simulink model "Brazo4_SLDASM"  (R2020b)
settings: Solver=VariableStepAuto  StartTime=0.0  StopTime=20  RelTol=1e-3
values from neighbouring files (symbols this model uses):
  q = [q 0]    [robotSimulation.m]    (also in robotSimulationWithConstraints.m = [q' 0])
undefined symbols (not defined in the file or in its folder): deg, kg, m, N, rad, s, X, Y, Z
libraries: sm_lib x118, nesl_utility x17, pid_lib x4
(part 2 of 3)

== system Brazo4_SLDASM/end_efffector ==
  Inertia : sm_lib/Body Elements/Inertia  InertiaType=Custom  Mass=1.4886  MassUnits=kg  CenterOfMass=[0, 0, 0]  CenterOfMassUnits=m  MomentsOfInertia=[0.00086527, 0.00086527, 0.0015073]  MomentsOfInertiaUnits=kg*m^2  ProductsOfInertia=[-1.4429e-20, -5.8421e-20, 3.3881e-21]  ProductsOfInertiaUnits=kg*m^2  GraphicType=None  MarkerShape=Inertia  MarkerSize=20  GraphicVisPropType=SimpleVisualProperties  GraphicDiffuseColor=[0.5 0.5 0.5]  GraphicSpecularColor=[0.5 0.5 0.5 1.0]  GraphicAmbientColor=[0.15 0.15 0.15 1.0]  GraphicEmissiveColor=[0.0 0.0 0.0 1.0]  GraphicShininess=75  GraphicOpacity=1.0
  InertiaOriginTransform : sm_lib/Frames and Transforms/Rigid Transform  TranslationMethod=Cartesian  TranslationStandardOffset=0  TranslationLengthUnit=m  TranslationStandardAxis=+Z  TranslationCartesianOffset=[5.5511e-17, -3.4694e-18, -0.015]  TranslationROffset=0  TranslationROffsetUnits=m  TranslationZOffset=0  TranslationZOffsetUnits=m  TranslationThetaOffset=0  TranslationThetaOffsetUnits=deg  RotationMethod=RotationSequence  RotationAngleUnits=deg  RotationStandardAxis=+Z  RotationAngle=0.0  RotationArbitraryAxis=[0 0 1]  FollAlignAxisA=+X  BaseAlignAxisA=+Y  FollAlignAxisB=+Y  BaseAlignAxisB=+Z  RotationSequenceAxes=BaseAxes  RotationSequence=XYZ  RotationSequenceAngles=[0, 0, 0]  RotationSequenceAnglesUnits=rad  RotationMatrix=[1 0 0; 0 1 0; 0 0 1]
  ReferenceFrame : sm_lib/Frames and Transforms/Reference Frame
  Visual : sm_lib/Body Elements/File Solid  ExtGeomFileName=Brazo4_SLDASM/meshes/end_efffector.STL  UnitType=Custom  ExtGeomFileUnits=m  StepReaderType=HEX  ExportConvexHullGeometry=off  InertiaType=Custom  Mass=0  MassUnits=kg  CenterOfMass=[0, 0, 0]  CenterOfMassUnits=m  MomentsOfInertia=[0, 0, 0]  MomentsOfInertiaUnits=kg*m^2  ProductsOfInertia=[0, 0, 0]  ProductsOfInertiaUnits=kg*m^2  BasedOnType=DensityFromFile  Density=1000  DensityUnits=kg/m^3  DoExposeReferenceFrame=on  SerializedFrames=<Frames/>  GraphicType=FromGeometry  MarkerShape=Sphere  MarkerSize=10  GraphicVisPropType=SimpleVisualProperties  GraphicDiffuseColor=[0.77647, 0.75686, 0.73725]  GraphicSpecularColor=[0.5 0.5 0.5 1.0]  GraphicAmbientColor=[0.15 0.15 0.15 1.0]  GraphicEmissiveColor=[0.0 0.0 0.0 1.0]  GraphicShininess=75  GraphicOpacity=1
  VisualOriginTransform : sm_lib/Frames and Transforms/Rigid Transform  TranslationMethod=Cartesian  TranslationStandardOffset=0  TranslationLengthUnit=m  TranslationStandardAxis=+Z  TranslationCartesianOffset=[0, 0, 0]  TranslationROffset=0  TranslationROffsetUnits=m  TranslationZOffset=0  TranslationZOffsetUnits=m  TranslationThetaOffset=0  TranslationThetaOffsetUnits=deg  RotationMethod=RotationSequence  RotationAngleUnits=deg  RotationStandardAxis=+Z  RotationAngle=0.0  RotationArbitraryAxis=[0 0 1]  FollAlignAxisA=+X  BaseAlignAxisA=+Y  FollAlignAxisB=+Y  BaseAlignAxisB=+Z  RotationSequenceAxes=BaseAxes  RotationSequence=XYZ  RotationSequenceAngles=[0, 0, 0]  RotationSequenceAnglesUnits=rad  RotationMatrix=[1 0 0; 0 1 0; 0 0 1]
  F : PMIOPort  Side=Left
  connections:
  Inertia/RConn1 -- InertiaOriginTransform/RConn1
  ReferenceFrame/RConn1 -- InertiaOriginTransform/LConn1 -- VisualOriginTransform/LConn1 -- F/RConn1
  Visual/RConn1 -- VisualOriginTransform/RConn1

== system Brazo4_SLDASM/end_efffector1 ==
  Inertia : sm_lib/Body Elements/Inertia  InertiaType=Custom  Mass=1.4886  MassUnits=kg  CenterOfMass=[0, 0, 0]  CenterOfMassUnits=m  MomentsOfInertia=[0.00086527, 0.00086527, 0.0015073]  MomentsOfInertiaUnits=kg*m^2  ProductsOfInertia=[-1.4429e-20, -5.8421e-20, 3.3881e-21]  ProductsOfInertiaUnits=kg*m^2  GraphicType=None  MarkerShape=Inertia  MarkerSize=20  GraphicVisPropType=SimpleVisualProperties  GraphicDiffuseColor=[0.5 0.5 0.5]  GraphicSpecularColor=[0.5 0.5 0.5 1.0]  GraphicAmbientColor=[0.15 0.15 0.15 1.0]  GraphicEmissiveColor=[0.0 0.0 0.0 1.0]  GraphicShininess=75  GraphicOpacity=1.0
  InertiaOriginTransform : sm_lib/Frames and Transforms/Rigid Transform  TranslationMethod=Cartesian  TranslationStandardOffset=0  TranslationLengthUnit=m  TranslationStandardAxis=+Z  TranslationCartesianOffset=[5.5511e-17, -3.4694e-18, -0.015]  TranslationROffset=0  TranslationROffsetUnits=m  TranslationZOffset=0  TranslationZOffsetUnits=m  TranslationThetaOffset=0  TranslationThetaOffsetUnits=deg  RotationMethod=RotationSequence  RotationAngleUnits=deg  RotationStandardAxis=+Z  RotationAngle=0.0  RotationArbitraryAxis=[0 0 1]  FollAlignAxisA=+X  BaseAlignAxisA=+Y  FollAlignAxisB=+Y  BaseAlignAxisB=+Z  RotationSequenceAxes=BaseAxes  RotationSequence=XYZ  RotationSequenceAngles=[0, 0, 0]  RotationSequenceAnglesUnits=rad  RotationMatrix=[1 0 0; 0 1 0; 0 0 1]
  ReferenceFrame : sm_lib/Frames and Transforms/Reference Frame
  Visual : sm_lib/Body Elements/File Solid  ExtGeomFileName=Brazo4_SLDASM/meshes/end_efffector.STL  UnitType=Custom  ExtGeomFileUnits=m  StepReaderType=HEX  ExportConvexHullGeometry=off  InertiaType=Custom  Mass=0  MassUnits=kg  CenterOfMass=[0, 0, 0]  CenterOfMassUnits=m  MomentsOfInertia=[0, 0, 0]  MomentsOfInertiaUnits=kg*m^2  ProductsOfInertia=[0, 0, 0]  ProductsOfInertiaUnits=kg*m^2  BasedOnType=DensityFromFile  Density=1000  DensityUnits=kg/m^3  DoExposeReferenceFrame=on  SerializedFrames=<Frames/>  GraphicType=FromGeometry  MarkerShape=Sphere  MarkerSize=10  GraphicVisPropType=SimpleVisualProperties  GraphicDiffuseColor=[0.77647, 0.75686, 0.73725]  GraphicSpecularColor=[0.5 0.5 0.5 1.0]  GraphicAmbientColor=[0.15 0.15 0.15 1.0]  GraphicEmissiveColor=[0.0 0.0 0.0 1.0]  GraphicShininess=75  GraphicOpacity=1
  VisualOriginTransform : sm_lib/Frames and Transforms/Rigid Transform  TranslationMethod=Cartesian  TranslationStandardOffset=0  TranslationLengthUnit=m  TranslationStandardAxis=+Z  TranslationCartesianOffset=[0, 0, 0]  TranslationROffset=0  TranslationROffsetUnits=m  TranslationZOffset=0  TranslationZOffsetUnits=m  TranslationThetaOffset=0  TranslationThetaOffsetUnits=deg  RotationMethod=RotationSequence  RotationAngleUnits=deg  RotationStandardAxis=+Z  RotationAngle=0.0  RotationArbitraryAxis=[0 0 1]  FollAlignAxisA=+X  BaseAlignAxisA=+Y  FollAlignAxisB=+Y  BaseAlignAxisB=+Z  RotationSequenceAxes=BaseAxes  RotationSequence=XYZ  RotationSequenceAngles=[0, 0, 0]  RotationSequenceAnglesUnits=rad  RotationMatrix=[1 0 0; 0 1 0; 0 0 1]
  F : PMIOPort  Side=Left
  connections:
  Inertia/RConn1 -- InertiaOriginTransform/RConn1
  ReferenceFrame/RConn1 -- InertiaOriginTransform/LConn1 -- VisualOriginTransform/LConn1 -- F/RConn1
  Visual/RConn1 -- VisualOriginTransform/RConn1

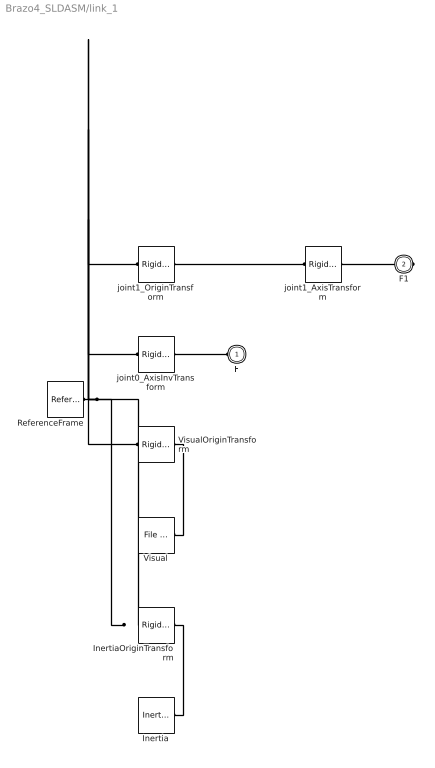
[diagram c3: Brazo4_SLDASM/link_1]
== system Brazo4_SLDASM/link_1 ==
  Inertia : sm_lib/Body Elements/Inertia  InertiaType=Custom  Mass=40.085  MassUnits=kg  CenterOfMass=[0, 0, 0]  CenterOfMassUnits=m  MomentsOfInertia=[0.14011, 0.15124, 0.16589]  MomentsOfInertiaUnits=kg*m^2  ProductsOfInertia=[-5.1752e-17, 1.3296e-17, 1.589e-18]  ProductsOfInertiaUnits=kg*m^2  GraphicType=None  MarkerShape=Inertia  MarkerSize=20  GraphicVisPropType=SimpleVisualProperties  GraphicDiffuseColor=[0.5 0.5 0.5]  GraphicSpecularColor=[0.5 0.5 0.5 1.0]  GraphicAmbientColor=[0.15 0.15 0.15 1.0]  GraphicEmissiveColor=[0.0 0.0 0.0 1.0]  GraphicShininess=75  GraphicOpacity=1.0
  InertiaOriginTransform : sm_lib/Frames and Transforms/Rigid Transform  TranslationMethod=Cartesian  TranslationStandardOffset=0  TranslationLengthUnit=m  TranslationStandardAxis=+Z  TranslationCartesianOffset=[2.7731e-17, 2.4685e-06, 0.28325]  TranslationROffset=0  TranslationROffsetUnits=m  TranslationZOffset=0  TranslationZOffsetUnits=m  TranslationThetaOffset=0  TranslationThetaOffsetUnits=deg  RotationMethod=RotationSequence  RotationAngleUnits=deg  RotationStandardAxis=+Z  RotationAngle=0.0  RotationArbitraryAxis=[0 0 1]  FollAlignAxisA=+X  BaseAlignAxisA=+Y  FollAlignAxisB=+Y  BaseAlignAxisB=+Z  RotationSequenceAxes=BaseAxes  RotationSequence=XYZ  RotationSequenceAngles=[0, 0, 0]  RotationSequenceAnglesUnits=rad  RotationMatrix=[1 0 0; 0 1 0; 0 0 1]
  ReferenceFrame : sm_lib/Frames and Transforms/Reference Frame
  Visual : sm_lib/Body Elements/File Solid  ExtGeomFileName=Brazo4_SLDASM/meshes/link_1.STL  UnitType=Custom  ExtGeomFileUnits=m  StepReaderType=HEX  ExportConvexHullGeometry=off  InertiaType=Custom  Mass=0  MassUnits=kg  CenterOfMass=[0, 0, 0]  CenterOfMassUnits=m  MomentsOfInertia=[0, 0, 0]  MomentsOfInertiaUnits=kg*m^2  ProductsOfInertia=[0, 0, 0]  ProductsOfInertiaUnits=kg*m^2  BasedOnType=DensityFromFile  Density=1000  DensityUnits=kg/m^3  DoExposeReferenceFrame=on  SerializedFrames=<Frames/>  GraphicType=FromGeometry  MarkerShape=Sphere  MarkerSize=10  GraphicVisPropType=SimpleVisualProperties  GraphicDiffuseColor=[0.77647, 0.75686, 0.73725]  GraphicSpecularColor=[0.5 0.5 0.5 1.0]  GraphicAmbientColor=[0.15 0.15 0.15 1.0]  GraphicEmissiveColor=[0.0 0.0 0.0 1.0]  GraphicShininess=75  GraphicOpacity=1
  VisualOriginTransform : sm_lib/Frames and Transforms/Rigid Transform  TranslationMethod=Cartesian  TranslationStandardOffset=0  TranslationLengthUnit=m  TranslationStandardAxis=+Z  TranslationCartesianOffset=[0, 0, 0]  TranslationROffset=0  TranslationROffsetUnits=m  TranslationZOffset=0  TranslationZOffsetUnits=m  TranslationThetaOffset=0  TranslationThetaOffsetUnits=deg  RotationMethod=RotationSequence  RotationAngleUnits=deg  RotationStandardAxis=+Z  RotationAngle=0.0  RotationArbitraryAxis=[0 0 1]  FollAlignAxisA=+X  BaseAlignAxisA=+Y  FollAlignAxisB=+Y  BaseAlignAxisB=+Z  RotationSequenceAxes=BaseAxes  RotationSequence=XYZ  RotationSequenceAngles=[0, 0, 0]  RotationSequenceAnglesUnits=rad  RotationMatrix=[1 0 0; 0 1 0; 0 0 1]
  joint0_AxisInvTransform : sm_lib/Frames and Transforms/Rigid Transform  TranslationMethod=Cartesian  TranslationStandardOffset=0  TranslationLengthUnit=m  TranslationStandardAxis=+Z  TranslationCartesianOffset=[0, 0, 0]  TranslationROffset=0  TranslationROffsetUnits=m  TranslationZOffset=0  TranslationZOffsetUnits=m  TranslationThetaOffset=0  TranslationThetaOffsetUnits=deg  RotationMethod=ArbitraryAxis  RotationAngleUnits=rad  RotationStandardAxis=+Z  RotationAngle=0  RotationArbitraryAxis=[1, 0, 0]  FollAlignAxisA=+X  BaseAlignAxisA=+Y  FollAlignAxisB=+Y  BaseAlignAxisB=+Z  RotationSequenceAxes=FollowerAxes  RotationSequence=XYX  RotationSequenceAngles=[0 0 0]  RotationSequenceAnglesUnits=deg  RotationMatrix=[1 0 0; 0 1 0; 0 0 1]
  joint1_AxisTransform : sm_lib/Frames and Transforms/Rigid Transform  TranslationMethod=Cartesian  TranslationStandardOffset=0  TranslationLengthUnit=m  TranslationStandardAxis=+Z  TranslationCartesianOffset=[0, 0, 0]  TranslationROffset=0  TranslationROffsetUnits=m  TranslationZOffset=0  TranslationZOffsetUnits=m  TranslationThetaOffset=0  TranslationThetaOffsetUnits=deg  RotationMethod=ArbitraryAxis  RotationAngleUnits=rad  RotationStandardAxis=+Z  RotationAngle=0  RotationArbitraryAxis=[1, 0, 0]  FollAlignAxisA=+X  BaseAlignAxisA=+Y  FollAlignAxisB=+Y  BaseAlignAxisB=+Z  RotationSequenceAxes=FollowerAxes  RotationSequence=XYX  RotationSequenceAngles=[0 0 0]  RotationSequenceAnglesUnits=deg  RotationMatrix=[1 0 0; 0 1 0; 0 0 1]
  joint1_OriginTransform : sm_lib/Frames and Transforms/Rigid Transform  TranslationMethod=Cartesian  TranslationStandardOffset=0  TranslationLengthUnit=m  TranslationStandardAxis=+Z  TranslationCartesianOffset=[0, 0, 0.35051]  TranslationROffset=0  TranslationROffsetUnits=m  TranslationZOffset=0  TranslationZOffsetUnits=m  TranslationThetaOffset=0  TranslationThetaOffsetUnits=deg  RotationMethod=RotationSequence  RotationAngleUnits=deg  RotationStandardAxis=+Z  RotationAngle=0.0  RotationArbitraryAxis=[0 0 1]  FollAlignAxisA=+X  BaseAlignAxisA=+Y  FollAlignAxisB=+Y  BaseAlignAxisB=+Z  RotationSequenceAxes=BaseAxes  RotationSequence=XYZ  RotationSequenceAngles=[1.5708, 0, 1.5708]  RotationSequenceAnglesUnits=rad  RotationMatrix=[1 0 0; 0 1 0; 0 0 1]
  F : PMIOPort  Side=Left
  F1 : PMIOPort  Port=2  Side=Right
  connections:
  Inertia/RConn1 -- InertiaOriginTransform/RConn1
  ReferenceFrame/RConn1 -- InertiaOriginTransform/LConn1 -- VisualOriginTransform/LConn1 -- joint0_AxisInvTransform/LConn1 -- joint1_OriginTransform/LConn1
  Visual/RConn1 -- VisualOriginTransform/RConn1
  joint0_AxisInvTransform/RConn1 -- F/RConn1
  joint1_AxisTransform/RConn1 -- F1/RConn1
  joint1_AxisTransform/LConn1 -- joint1_OriginTransform/RConn1

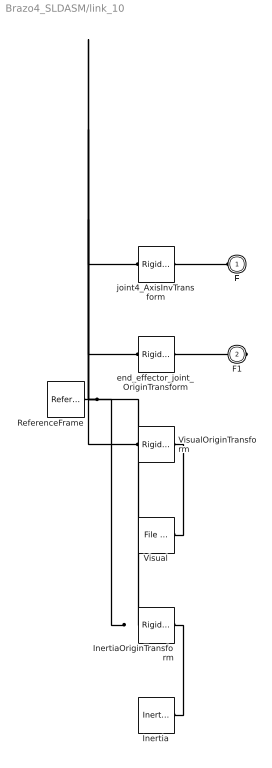
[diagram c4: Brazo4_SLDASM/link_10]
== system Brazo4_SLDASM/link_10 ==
  Inertia : sm_lib/Body Elements/Inertia  InertiaType=Custom  Mass=1.4886  MassUnits=kg  CenterOfMass=[0, 0, 0]  CenterOfMassUnits=m  MomentsOfInertia=[0.00086527, 0.00086527, 0.0015073]  MomentsOfInertiaUnits=kg*m^2  ProductsOfInertia=[-1.5349e-20, -1.2683e-19, -7.4327e-21]  ProductsOfInertiaUnits=kg*m^2  GraphicType=None  MarkerShape=Inertia  MarkerSize=20  GraphicVisPropType=SimpleVisualProperties  GraphicDiffuseColor=[0.5 0.5 0.5]  GraphicSpecularColor=[0.5 0.5 0.5 1.0]  GraphicAmbientColor=[0.15 0.15 0.15 1.0]  GraphicEmissiveColor=[0.0 0.0 0.0 1.0]  GraphicShininess=75  GraphicOpacity=1.0
  InertiaOriginTransform : sm_lib/Frames and Transforms/Rigid Transform  TranslationMethod=Cartesian  TranslationStandardOffset=0  TranslationLengthUnit=m  TranslationStandardAxis=+Z  TranslationCartesianOffset=[1.1102e-16, -1.5173e-17, 0.08550000000000001]  TranslationROffset=0  TranslationROffsetUnits=m  TranslationZOffset=0  TranslationZOffsetUnits=m  TranslationThetaOffset=0  TranslationThetaOffsetUnits=deg  RotationMethod=RotationSequence  RotationAngleUnits=deg  RotationStandardAxis=+Z  RotationAngle=0.0  RotationArbitraryAxis=[0 0 1]  FollAlignAxisA=+X  BaseAlignAxisA=+Y  FollAlignAxisB=+Y  BaseAlignAxisB=+Z  RotationSequenceAxes=BaseAxes  RotationSequence=XYZ  RotationSequenceAngles=[0, 0, 0]  RotationSequenceAnglesUnits=rad  RotationMatrix=[1 0 0; 0 1 0; 0 0 1]
  ReferenceFrame : sm_lib/Frames and Transforms/Reference Frame
  Visual : sm_lib/Body Elements/File Solid  ExtGeomFileName=Brazo4_SLDASM/meshes/link_5.STL  UnitType=Custom  ExtGeomFileUnits=m  StepReaderType=HEX  ExportConvexHullGeometry=off  InertiaType=Custom  Mass=0  MassUnits=kg  CenterOfMass=[0, 0, 0]  CenterOfMassUnits=m  MomentsOfInertia=[0, 0, 0]  MomentsOfInertiaUnits=kg*m^2  ProductsOfInertia=[0, 0, 0]  ProductsOfInertiaUnits=kg*m^2  BasedOnType=DensityFromFile  Density=1000  DensityUnits=kg/m^3  DoExposeReferenceFrame=on  SerializedFrames=<Frames/>  GraphicType=FromGeometry  MarkerShape=Sphere  MarkerSize=10  GraphicVisPropType=SimpleVisualProperties  GraphicDiffuseColor=[0.77647, 0.75686, 0.73725]  GraphicSpecularColor=[0.5 0.5 0.5 1.0]  GraphicAmbientColor=[0.15 0.15 0.15 1.0]  GraphicEmissiveColor=[0.0 0.0 0.0 1.0]  GraphicShininess=75  GraphicOpacity=1
  VisualOriginTransform : sm_lib/Frames and Transforms/Rigid Transform  TranslationMethod=Cartesian  TranslationStandardOffset=0  TranslationLengthUnit=m  TranslationStandardAxis=+Z  TranslationCartesianOffset=[0, 0, 0]  TranslationROffset=0  TranslationROffsetUnits=m  TranslationZOffset=0  TranslationZOffsetUnits=m  TranslationThetaOffset=0  TranslationThetaOffsetUnits=deg  RotationMethod=RotationSequence  RotationAngleUnits=deg  RotationStandardAxis=+Z  RotationAngle=0.0  RotationArbitraryAxis=[0 0 1]  FollAlignAxisA=+X  BaseAlignAxisA=+Y  FollAlignAxisB=+Y  BaseAlignAxisB=+Z  RotationSequenceAxes=BaseAxes  RotationSequence=XYZ  RotationSequenceAngles=[0, 0, 0]  RotationSequenceAnglesUnits=rad  RotationMatrix=[1 0 0; 0 1 0; 0 0 1]
  end_effector_joint_OriginTransform : sm_lib/Frames and Transforms/Rigid Transform  TranslationMethod=Cartesian  TranslationStandardOffset=0  TranslationLengthUnit=m  TranslationStandardAxis=+Z  TranslationCartesianOffset=[0, 0, 0.1005]  TranslationROffset=0  TranslationROffsetUnits=m  TranslationZOffset=0  TranslationZOffsetUnits=m  TranslationThetaOffset=0  TranslationThetaOffsetUnits=deg  RotationMethod=RotationSequence  RotationAngleUnits=deg  RotationStandardAxis=+Z  RotationAngle=0.0  RotationArbitraryAxis=[0 0 1]  FollAlignAxisA=+X  BaseAlignAxisA=+Y  FollAlignAxisB=+Y  BaseAlignAxisB=+Z  RotationSequenceAxes=BaseAxes  RotationSequence=XYZ  RotationSequenceAngles=[0, 0, 0.045381]  RotationSequenceAnglesUnits=rad  RotationMatrix=[1 0 0; 0 1 0; 0 0 1]
  joint4_AxisInvTransform : sm_lib/Frames and Transforms/Rigid Transform  TranslationMethod=Cartesian  TranslationStandardOffset=0  TranslationLengthUnit=m  TranslationStandardAxis=+Z  TranslationCartesianOffset=[0, 0, 0]  TranslationROffset=0  TranslationROffsetUnits=m  TranslationZOffset=0  TranslationZOffsetUnits=m  TranslationThetaOffset=0  TranslationThetaOffsetUnits=deg  RotationMethod=ArbitraryAxis  RotationAngleUnits=rad  RotationStandardAxis=+Z  RotationAngle=0  RotationArbitraryAxis=[1, 0, 0]  FollAlignAxisA=+X  BaseAlignAxisA=+Y  FollAlignAxisB=+Y  BaseAlignAxisB=+Z  RotationSequenceAxes=FollowerAxes  RotationSequence=XYX  RotationSequenceAngles=[0 0 0]  RotationSequenceAnglesUnits=deg  RotationMatrix=[1 0 0; 0 1 0; 0 0 1]
  F : PMIOPort  Side=Left
  F1 : PMIOPort  Port=2  Side=Right
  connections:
  Inertia/RConn1 -- InertiaOriginTransform/RConn1
  ReferenceFrame/RConn1 -- InertiaOriginTransform/LConn1 -- VisualOriginTransform/LConn1 -- end_effector_joint_OriginTransform/LConn1 -- joint4_AxisInvTransform/LConn1
  Visual/RConn1 -- VisualOriginTransform/RConn1
  end_effector_joint_OriginTransform/RConn1 -- F1/RConn1
  joint4_AxisInvTransform/RConn1 -- F/RConn1

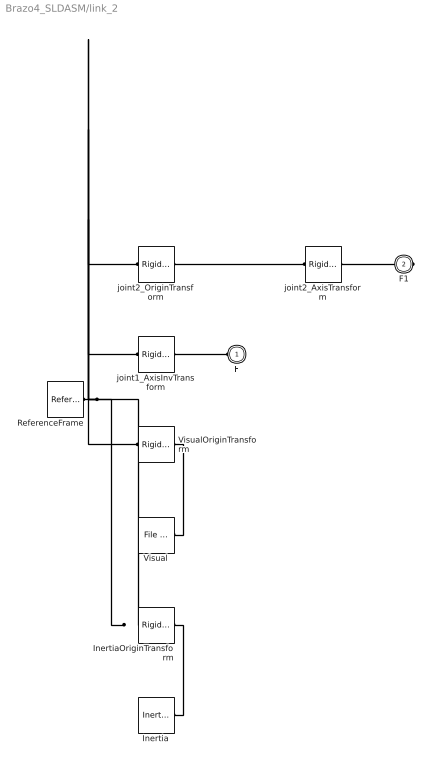
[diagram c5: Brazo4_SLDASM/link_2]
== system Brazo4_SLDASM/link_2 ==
  Inertia : sm_lib/Body Elements/Inertia  InertiaType=Custom  Mass=34.189  MassUnits=kg  CenterOfMass=[0, 0, 0]  CenterOfMassUnits=m  MomentsOfInertia=[0.101, 0.32346, 0.28584]  MomentsOfInertiaUnits=kg*m^2  ProductsOfInertia=[-2.191e-18, 8.7345e-17, 3.6996e-17]  ProductsOfInertiaUnits=kg*m^2  GraphicType=None  MarkerShape=Inertia  MarkerSize=20  GraphicVisPropType=SimpleVisualProperties  GraphicDiffuseColor=[0.5 0.5 0.5]  GraphicSpecularColor=[0.5 0.5 0.5 1.0]  GraphicAmbientColor=[0.15 0.15 0.15 1.0]  GraphicEmissiveColor=[0.0 0.0 0.0 1.0]  GraphicShininess=75  GraphicOpacity=1.0
  InertiaOriginTransform : sm_lib/Frames and Transforms/Rigid Transform  TranslationMethod=Cartesian  TranslationStandardOffset=0  TranslationLengthUnit=m  TranslationStandardAxis=+Z  TranslationCartesianOffset=[0.07391200000000001, 0, -1.2748e-17]  TranslationROffset=0  TranslationROffsetUnits=m  TranslationZOffset=0  TranslationZOffsetUnits=m  TranslationThetaOffset=0  TranslationThetaOffsetUnits=deg  RotationMethod=RotationSequence  RotationAngleUnits=deg  RotationStandardAxis=+Z  RotationAngle=0.0  RotationArbitraryAxis=[0 0 1]  FollAlignAxisA=+X  BaseAlignAxisA=+Y  FollAlignAxisB=+Y  BaseAlignAxisB=+Z  RotationSequenceAxes=BaseAxes  RotationSequence=XYZ  RotationSequenceAngles=[0, 0, 0]  RotationSequenceAnglesUnits=rad  RotationMatrix=[1 0 0; 0 1 0; 0 0 1]
  ReferenceFrame : sm_lib/Frames and Transforms/Reference Frame
  Visual : sm_lib/Body Elements/File Solid  ExtGeomFileName=Brazo4_SLDASM/meshes/link_2.STL  UnitType=Custom  ExtGeomFileUnits=m  StepReaderType=HEX  ExportConvexHullGeometry=off  InertiaType=Custom  Mass=0  MassUnits=kg  CenterOfMass=[0, 0, 0]  CenterOfMassUnits=m  MomentsOfInertia=[0, 0, 0]  MomentsOfInertiaUnits=kg*m^2  ProductsOfInertia=[0, 0, 0]  ProductsOfInertiaUnits=kg*m^2  BasedOnType=DensityFromFile  Density=1000  DensityUnits=kg/m^3  DoExposeReferenceFrame=on  SerializedFrames=<Frames/>  GraphicType=FromGeometry  MarkerShape=Sphere  MarkerSize=10  GraphicVisPropType=SimpleVisualProperties  GraphicDiffuseColor=[0.77647, 0.75686, 0.73725]  GraphicSpecularColor=[0.5 0.5 0.5 1.0]  GraphicAmbientColor=[0.15 0.15 0.15 1.0]  GraphicEmissiveColor=[0.0 0.0 0.0 1.0]  GraphicShininess=75  GraphicOpacity=1
  VisualOriginTransform : sm_lib/Frames and Transforms/Rigid Transform  TranslationMethod=Cartesian  TranslationStandardOffset=0  TranslationLengthUnit=m  TranslationStandardAxis=+Z  TranslationCartesianOffset=[0, 0, 0]  TranslationROffset=0  TranslationROffsetUnits=m  TranslationZOffset=0  TranslationZOffsetUnits=m  TranslationThetaOffset=0  TranslationThetaOffsetUnits=deg  RotationMethod=RotationSequence  RotationAngleUnits=deg  RotationStandardAxis=+Z  RotationAngle=0.0  RotationArbitraryAxis=[0 0 1]  FollAlignAxisA=+X  BaseAlignAxisA=+Y  FollAlignAxisB=+Y  BaseAlignAxisB=+Z  RotationSequenceAxes=BaseAxes  RotationSequence=XYZ  RotationSequenceAngles=[0, 0, 0]  RotationSequenceAnglesUnits=rad  RotationMatrix=[1 0 0; 0 1 0; 0 0 1]
  joint1_AxisInvTransform : sm_lib/Frames and Transforms/Rigid Transform  TranslationMethod=Cartesian  TranslationStandardOffset=0  TranslationLengthUnit=m  TranslationStandardAxis=+Z  TranslationCartesianOffset=[0, 0, 0]  TranslationROffset=0  TranslationROffsetUnits=m  TranslationZOffset=0  TranslationZOffsetUnits=m  TranslationThetaOffset=0  TranslationThetaOffsetUnits=deg  RotationMethod=ArbitraryAxis  RotationAngleUnits=rad  RotationStandardAxis=+Z  RotationAngle=0  RotationArbitraryAxis=[1, 0, 0]  FollAlignAxisA=+X  BaseAlignAxisA=+Y  FollAlignAxisB=+Y  BaseAlignAxisB=+Z  RotationSequenceAxes=FollowerAxes  RotationSequence=XYX  RotationSequenceAngles=[0 0 0]  RotationSequenceAnglesUnits=deg  RotationMatrix=[1 0 0; 0 1 0; 0 0 1]
  joint2_AxisTransform : sm_lib/Frames and Transforms/Rigid Transform  TranslationMethod=Cartesian  TranslationStandardOffset=0  TranslationLengthUnit=m  TranslationStandardAxis=+Z  TranslationCartesianOffset=[0, 0, 0]  TranslationROffset=0  TranslationROffsetUnits=m  TranslationZOffset=0  TranslationZOffsetUnits=m  TranslationThetaOffset=0  TranslationThetaOffsetUnits=deg  RotationMethod=ArbitraryAxis  RotationAngleUnits=rad  RotationStandardAxis=+Z  RotationAngle=0  RotationArbitraryAxis=[1, 0, 0]  FollAlignAxisA=+X  BaseAlignAxisA=+Y  FollAlignAxisB=+Y  BaseAlignAxisB=+Z  RotationSequenceAxes=FollowerAxes  RotationSequence=XYX  RotationSequenceAngles=[0 0 0]  RotationSequenceAnglesUnits=deg  RotationMatrix=[1 0 0; 0 1 0; 0 0 1]
  joint2_OriginTransform : sm_lib/Frames and Transforms/Rigid Transform  TranslationMethod=Cartesian  TranslationStandardOffset=0  TranslationLengthUnit=m  TranslationStandardAxis=+Z  TranslationCartesianOffset=[0.25, 0, 0]  TranslationROffset=0  TranslationROffsetUnits=m  TranslationZOffset=0  TranslationZOffsetUnits=m  TranslationThetaOffset=0  TranslationThetaOffsetUnits=deg  RotationMethod=RotationSequence  RotationAngleUnits=deg  RotationStandardAxis=+Z  RotationAngle=0.0  RotationArbitraryAxis=[0 0 1]  FollAlignAxisA=+X  BaseAlignAxisA=+Y  FollAlignAxisB=+Y  BaseAlignAxisB=+Z  RotationSequenceAxes=BaseAxes  RotationSequence=XYZ  RotationSequenceAngles=[0, 0, 0]  RotationSequenceAnglesUnits=rad  RotationMatrix=[1 0 0; 0 1 0; 0 0 1]
  F : PMIOPort  Side=Left
  F1 : PMIOPort  Port=2  Side=Right
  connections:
  Inertia/RConn1 -- InertiaOriginTransform/RConn1
  ReferenceFrame/RConn1 -- InertiaOriginTransform/LConn1 -- VisualOriginTransform/LConn1 -- joint1_AxisInvTransform/LConn1 -- joint2_OriginTransform/LConn1
  Visual/RConn1 -- VisualOriginTransform/RConn1
  joint1_AxisInvTransform/RConn1 -- F/RConn1
  joint2_AxisTransform/RConn1 -- F1/RConn1
  joint2_AxisTransform/LConn1 -- joint2_OriginTransform/RConn1

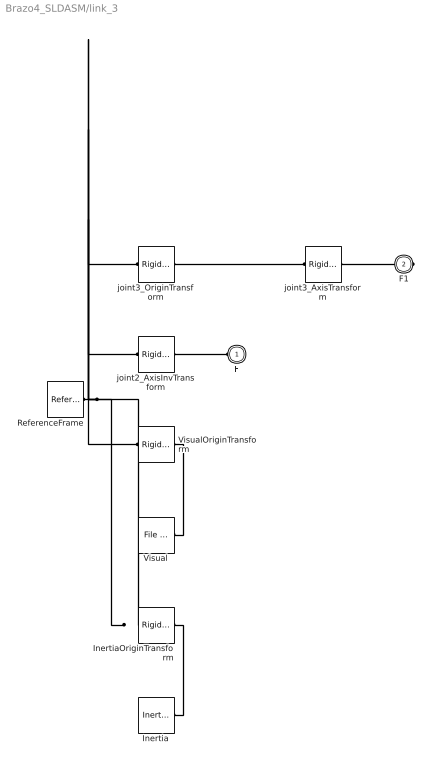
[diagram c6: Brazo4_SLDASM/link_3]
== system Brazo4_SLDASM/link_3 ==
  Inertia : sm_lib/Body Elements/Inertia  InertiaType=Custom  Mass=13.946  MassUnits=kg  CenterOfMass=[0, 0, 0]  CenterOfMassUnits=m  MomentsOfInertia=[0.026465, 0.06281399999999999, 0.054336]  MomentsOfInertiaUnits=kg*m^2  ProductsOfInertia=[-5.1463e-19, 1.9268e-17, 6.4193e-18]  ProductsOfInertiaUnits=kg*m^2  GraphicType=None  MarkerShape=Inertia  MarkerSize=20  GraphicVisPropType=SimpleVisualProperties  GraphicDiffuseColor=[0.5 0.5 0.5]  GraphicSpecularColor=[0.5 0.5 0.5 1.0]  GraphicAmbientColor=[0.15 0.15 0.15 1.0]  GraphicEmissiveColor=[0.0 0.0 0.0 1.0]  GraphicShininess=75  GraphicOpacity=1.0
  InertiaOriginTransform : sm_lib/Frames and Transforms/Rigid Transform  TranslationMethod=Cartesian  TranslationStandardOffset=0  TranslationLengthUnit=m  TranslationStandardAxis=+Z  TranslationCartesianOffset=[0.053841, 0, -3.1131e-17]  TranslationROffset=0  TranslationROffsetUnits=m  TranslationZOffset=0  TranslationZOffsetUnits=m  TranslationThetaOffset=0  TranslationThetaOffsetUnits=deg  RotationMethod=RotationSequence  RotationAngleUnits=deg  RotationStandardAxis=+Z  RotationAngle=0.0  RotationArbitraryAxis=[0 0 1]  FollAlignAxisA=+X  BaseAlignAxisA=+Y  FollAlignAxisB=+Y  BaseAlignAxisB=+Z  RotationSequenceAxes=BaseAxes  RotationSequence=XYZ  RotationSequenceAngles=[0, 0, 0]  RotationSequenceAnglesUnits=rad  RotationMatrix=[1 0 0; 0 1 0; 0 0 1]
  ReferenceFrame : sm_lib/Frames and Transforms/Reference Frame
  Visual : sm_lib/Body Elements/File Solid  ExtGeomFileName=Brazo4_SLDASM/meshes/link_3.STL  UnitType=Custom  ExtGeomFileUnits=m  StepReaderType=HEX  ExportConvexHullGeometry=off  InertiaType=Custom  Mass=0  MassUnits=kg  CenterOfMass=[0, 0, 0]  CenterOfMassUnits=m  MomentsOfInertia=[0, 0, 0]  MomentsOfInertiaUnits=kg*m^2  ProductsOfInertia=[0, 0, 0]  ProductsOfInertiaUnits=kg*m^2  BasedOnType=DensityFromFile  Density=1000  DensityUnits=kg/m^3  DoExposeReferenceFrame=on  SerializedFrames=<Frames/>  GraphicType=FromGeometry  MarkerShape=Sphere  MarkerSize=10  GraphicVisPropType=SimpleVisualProperties  GraphicDiffuseColor=[0.77647, 0.75686, 0.73725]  GraphicSpecularColor=[0.5 0.5 0.5 1.0]  GraphicAmbientColor=[0.15 0.15 0.15 1.0]  GraphicEmissiveColor=[0.0 0.0 0.0 1.0]  GraphicShininess=75  GraphicOpacity=1
  VisualOriginTransform : sm_lib/Frames and Transforms/Rigid Transform  TranslationMethod=Cartesian  TranslationStandardOffset=0  TranslationLengthUnit=m  TranslationStandardAxis=+Z  TranslationCartesianOffset=[0, 0, 0]  TranslationROffset=0  TranslationROffsetUnits=m  TranslationZOffset=0  TranslationZOffsetUnits=m  TranslationThetaOffset=0  TranslationThetaOffsetUnits=deg  RotationMethod=RotationSequence  RotationAngleUnits=deg  RotationStandardAxis=+Z  RotationAngle=0.0  RotationArbitraryAxis=[0 0 1]  FollAlignAxisA=+X  BaseAlignAxisA=+Y  FollAlignAxisB=+Y  BaseAlignAxisB=+Z  RotationSequenceAxes=BaseAxes  RotationSequence=XYZ  RotationSequenceAngles=[0, 0, 0]  RotationSequenceAnglesUnits=rad  RotationMatrix=[1 0 0; 0 1 0; 0 0 1]
  joint2_AxisInvTransform : sm_lib/Frames and Transforms/Rigid Transform  TranslationMethod=Cartesian  TranslationStandardOffset=0  TranslationLengthUnit=m  TranslationStandardAxis=+Z  TranslationCartesianOffset=[0, 0, 0]  TranslationROffset=0  TranslationROffsetUnits=m  TranslationZOffset=0  TranslationZOffsetUnits=m  TranslationThetaOffset=0  TranslationThetaOffsetUnits=deg  RotationMethod=ArbitraryAxis  RotationAngleUnits=rad  RotationStandardAxis=+Z  RotationAngle=0  RotationArbitraryAxis=[1, 0, 0]  FollAlignAxisA=+X  BaseAlignAxisA=+Y  FollAlignAxisB=+Y  BaseAlignAxisB=+Z  RotationSequenceAxes=FollowerAxes  RotationSequence=XYX  RotationSequenceAngles=[0 0 0]  RotationSequenceAnglesUnits=deg  RotationMatrix=[1 0 0; 0 1 0; 0 0 1]
  joint3_AxisTransform : sm_lib/Frames and Transforms/Rigid Transform  TranslationMethod=Cartesian  TranslationStandardOffset=0  TranslationLengthUnit=m  TranslationStandardAxis=+Z  TranslationCartesianOffset=[0, 0, 0]  TranslationROffset=0  TranslationROffsetUnits=m  TranslationZOffset=0  TranslationZOffsetUnits=m  TranslationThetaOffset=0  TranslationThetaOffsetUnits=deg  RotationMethod=ArbitraryAxis  RotationAngleUnits=rad  RotationStandardAxis=+Z  RotationAngle=0  RotationArbitraryAxis=[1, 0, 0]  FollAlignAxisA=+X  BaseAlignAxisA=+Y  FollAlignAxisB=+Y  BaseAlignAxisB=+Z  RotationSequenceAxes=FollowerAxes  RotationSequence=XYX  RotationSequenceAngles=[0 0 0]  RotationSequenceAnglesUnits=deg  RotationMatrix=[1 0 0; 0 1 0; 0 0 1]
  joint3_OriginTransform : sm_lib/Frames and Transforms/Rigid Transform  TranslationMethod=Cartesian  TranslationStandardOffset=0  TranslationLengthUnit=m  TranslationStandardAxis=+Z  TranslationCartesianOffset=[0.16, 0, 0]  TranslationROffset=0  TranslationROffsetUnits=m  TranslationZOffset=0  TranslationZOffsetUnits=m  TranslationThetaOffset=0  TranslationThetaOffsetUnits=deg  RotationMethod=RotationSequence  RotationAngleUnits=deg  RotationStandardAxis=+Z  RotationAngle=0.0  RotationArbitraryAxis=[0 0 1]  FollAlignAxisA=+X  BaseAlignAxisA=+Y  FollAlignAxisB=+Y  BaseAlignAxisB=+Z  RotationSequenceAxes=BaseAxes  RotationSequence=XYZ  RotationSequenceAngles=[0, 0, 0]  RotationSequenceAnglesUnits=rad  RotationMatrix=[1 0 0; 0 1 0; 0 0 1]
  F : PMIOPort  Side=Left
  F1 : PMIOPort  Port=2  Side=Right
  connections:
  Inertia/RConn1 -- InertiaOriginTransform/RConn1
  ReferenceFrame/RConn1 -- InertiaOriginTransform/LConn1 -- VisualOriginTransform/LConn1 -- joint2_AxisInvTransform/LConn1 -- joint3_OriginTransform/LConn1
  Visual/RConn1 -- VisualOriginTransform/RConn1
  joint2_AxisInvTransform/RConn1 -- F/RConn1
  joint3_AxisTransform/RConn1 -- F1/RConn1
  joint3_AxisTransform/LConn1 -- joint3_OriginTransform/RConn1

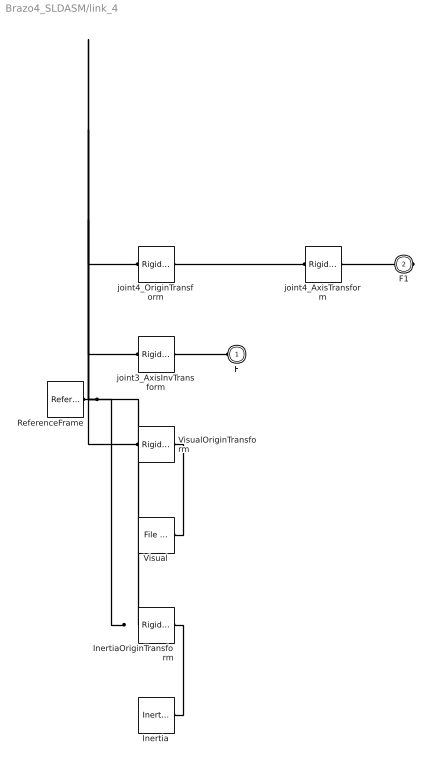
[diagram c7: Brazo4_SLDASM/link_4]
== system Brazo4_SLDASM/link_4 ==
  Inertia : sm_lib/Body Elements/Inertia  InertiaType=Custom  Mass=2.6258  MassUnits=kg  CenterOfMass=[0, 0, 0]  CenterOfMassUnits=m  MomentsOfInertia=[0.0019708, 0.0032587, 0.0021473]  MomentsOfInertiaUnits=kg*m^2  ProductsOfInertia=[-1.2627e-19, -3.1081e-19, 2.4201e-20]  ProductsOfInertiaUnits=kg*m^2  GraphicType=None  MarkerShape=Inertia  MarkerSize=20  GraphicVisPropType=SimpleVisualProperties  GraphicDiffuseColor=[0.5 0.5 0.5]  GraphicSpecularColor=[0.5 0.5 0.5 1.0]  GraphicAmbientColor=[0.15 0.15 0.15 1.0]  GraphicEmissiveColor=[0.0 0.0 0.0 1.0]  GraphicShininess=75  GraphicOpacity=1.0
  InertiaOriginTransform : sm_lib/Frames and Transforms/Rigid Transform  TranslationMethod=Cartesian  TranslationStandardOffset=0  TranslationLengthUnit=m  TranslationStandardAxis=+Z  TranslationCartesianOffset=[0.026026, -5.5511e-17, 3.1752e-17]  TranslationROffset=0  TranslationROffsetUnits=m  TranslationZOffset=0  TranslationZOffsetUnits=m  TranslationThetaOffset=0  TranslationThetaOffsetUnits=deg  RotationMethod=RotationSequence  RotationAngleUnits=deg  RotationStandardAxis=+Z  RotationAngle=0.0  RotationArbitraryAxis=[0 0 1]  FollAlignAxisA=+X  BaseAlignAxisA=+Y  FollAlignAxisB=+Y  BaseAlignAxisB=+Z  RotationSequenceAxes=BaseAxes  RotationSequence=XYZ  RotationSequenceAngles=[0, 0, 0]  RotationSequenceAnglesUnits=rad  RotationMatrix=[1 0 0; 0 1 0; 0 0 1]
  ReferenceFrame : sm_lib/Frames and Transforms/Reference Frame
  Visual : sm_lib/Body Elements/File Solid  ExtGeomFileName=Brazo4_SLDASM/meshes/link_4.STL  UnitType=Custom  ExtGeomFileUnits=m  StepReaderType=HEX  ExportConvexHullGeometry=off  InertiaType=Custom  Mass=0  MassUnits=kg  CenterOfMass=[0, 0, 0]  CenterOfMassUnits=m  MomentsOfInertia=[0, 0, 0]  MomentsOfInertiaUnits=kg*m^2  ProductsOfInertia=[0, 0, 0]  ProductsOfInertiaUnits=kg*m^2  BasedOnType=DensityFromFile  Density=1000  DensityUnits=kg/m^3  DoExposeReferenceFrame=on  SerializedFrames=<Frames/>  GraphicType=FromGeometry  MarkerShape=Sphere  MarkerSize=10  GraphicVisPropType=SimpleVisualProperties  GraphicDiffuseColor=[0.77647, 0.75686, 0.73725]  GraphicSpecularColor=[0.5 0.5 0.5 1.0]  GraphicAmbientColor=[0.15 0.15 0.15 1.0]  GraphicEmissiveColor=[0.0 0.0 0.0 1.0]  GraphicShininess=75  GraphicOpacity=1
  VisualOriginTransform : sm_lib/Frames and Transforms/Rigid Transform  TranslationMethod=Cartesian  TranslationStandardOffset=0  TranslationLengthUnit=m  TranslationStandardAxis=+Z  TranslationCartesianOffset=[0, 0, 0]  TranslationROffset=0  TranslationROffsetUnits=m  TranslationZOffset=0  TranslationZOffsetUnits=m  TranslationThetaOffset=0  TranslationThetaOffsetUnits=deg  RotationMethod=RotationSequence  RotationAngleUnits=deg  RotationStandardAxis=+Z  RotationAngle=0.0  RotationArbitraryAxis=[0 0 1]  FollAlignAxisA=+X  BaseAlignAxisA=+Y  FollAlignAxisB=+Y  BaseAlignAxisB=+Z  RotationSequenceAxes=BaseAxes  RotationSequence=XYZ  RotationSequenceAngles=[0, 0, 0]  RotationSequenceAnglesUnits=rad  RotationMatrix=[1 0 0; 0 1 0; 0 0 1]
  joint3_AxisInvTransform : sm_lib/Frames and Transforms/Rigid Transform  TranslationMethod=Cartesian  TranslationStandardOffset=0  TranslationLengthUnit=m  TranslationStandardAxis=+Z  TranslationCartesianOffset=[0, 0, 0]  TranslationROffset=0  TranslationROffsetUnits=m  TranslationZOffset=0  TranslationZOffsetUnits=m  TranslationThetaOffset=0  TranslationThetaOffsetUnits=deg  RotationMethod=ArbitraryAxis  RotationAngleUnits=rad  RotationStandardAxis=+Z  RotationAngle=0  RotationArbitraryAxis=[1, 0, 0]  FollAlignAxisA=+X  BaseAlignAxisA=+Y  FollAlignAxisB=+Y  BaseAlignAxisB=+Z  RotationSequenceAxes=FollowerAxes  RotationSequence=XYX  RotationSequenceAngles=[0 0 0]  RotationSequenceAnglesUnits=deg  RotationMatrix=[1 0 0; 0 1 0; 0 0 1]
  joint4_AxisTransform : sm_lib/Frames and Transforms/Rigid Transform  TranslationMethod=Cartesian  TranslationStandardOffset=0  TranslationLengthUnit=m  TranslationStandardAxis=+Z  TranslationCartesianOffset=[0, 0, 0]  TranslationROffset=0  TranslationROffsetUnits=m  TranslationZOffset=0  TranslationZOffsetUnits=m  TranslationThetaOffset=0  TranslationThetaOffsetUnits=deg  RotationMethod=ArbitraryAxis  RotationAngleUnits=rad  RotationStandardAxis=+Z  RotationAngle=0  RotationArbitraryAxis=[1, 0, 0]  FollAlignAxisA=+X  BaseAlignAxisA=+Y  FollAlignAxisB=+Y  BaseAlignAxisB=+Z  RotationSequenceAxes=FollowerAxes  RotationSequence=XYX  RotationSequenceAngles=[0 0 0]  RotationSequenceAnglesUnits=deg  RotationMatrix=[1 0 0; 0 1 0; 0 0 1]
  joint4_OriginTransform : sm_lib/Frames and Transforms/Rigid Transform  TranslationMethod=Cartesian  TranslationStandardOffset=0  TranslationLengthUnit=m  TranslationStandardAxis=+Z  TranslationCartesianOffset=[0, 0, 0]  TranslationROffset=0  TranslationROffsetUnits=m  TranslationZOffset=0  TranslationZOffsetUnits=m  TranslationThetaOffset=0  TranslationThetaOffsetUnits=deg  RotationMethod=RotationSequence  RotationAngleUnits=deg  RotationStandardAxis=+Z  RotationAngle=0.0  RotationArbitraryAxis=[0 0 1]  FollAlignAxisA=+X  BaseAlignAxisA=+Y  FollAlignAxisB=+Y  BaseAlignAxisB=+Z  RotationSequenceAxes=BaseAxes  RotationSequence=XYZ  RotationSequenceAngles=[1.5708, 0, 1.5708]  RotationSequenceAnglesUnits=rad  RotationMatrix=[1 0 0; 0 1 0; 0 0 1]
  F : PMIOPort  Side=Left
  F1 : PMIOPort  Port=2  Side=Right
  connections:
  Inertia/RConn1 -- InertiaOriginTransform/RConn1
  ReferenceFrame/RConn1 -- InertiaOriginTransform/LConn1 -- VisualOriginTransform/LConn1 -- joint3_AxisInvTransform/LConn1 -- joint4_OriginTransform/LConn1
  Visual/RConn1 -- VisualOriginTransform/RConn1
  joint3_AxisInvTransform/RConn1 -- F/RConn1
  joint4_AxisTransform/RConn1 -- F1/RConn1
  joint4_AxisTransform/LConn1 -- joint4_OriginTransform/RConn1

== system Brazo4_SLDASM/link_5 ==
  Inertia : sm_lib/Body Elements/Inertia  InertiaType=Custom  Mass=1.4886  MassUnits=kg  CenterOfMass=[0, 0, 0]  CenterOfMassUnits=m  MomentsOfInertia=[0.00086527, 0.00086527, 0.0015073]  MomentsOfInertiaUnits=kg*m^2  ProductsOfInertia=[-1.5349e-20, -1.2683e-19, -7.4327e-21]  ProductsOfInertiaUnits=kg*m^2  GraphicType=None  MarkerShape=Inertia  MarkerSize=20  GraphicVisPropType=SimpleVisualProperties  GraphicDiffuseColor=[0.5 0.5 0.5]  GraphicSpecularColor=[0.5 0.5 0.5 1.0]  GraphicAmbientColor=[0.15 0.15 0.15 1.0]  GraphicEmissiveColor=[0.0 0.0 0.0 1.0]  GraphicShininess=75  GraphicOpacity=1.0
  InertiaOriginTransform : sm_lib/Frames and Transforms/Rigid Transform  TranslationMethod=Cartesian  TranslationStandardOffset=0  TranslationLengthUnit=m  TranslationStandardAxis=+Z  TranslationCartesianOffset=[1.1102e-16, -1.5173e-17, 0.08550000000000001]  TranslationROffset=0  TranslationROffsetUnits=m  TranslationZOffset=0  TranslationZOffsetUnits=m  TranslationThetaOffset=0  TranslationThetaOffsetUnits=deg  RotationMethod=RotationSequence  RotationAngleUnits=deg  RotationStandardAxis=+Z  RotationAngle=0.0  RotationArbitraryAxis=[0 0 1]  FollAlignAxisA=+X  BaseAlignAxisA=+Y  FollAlignAxisB=+Y  BaseAlignAxisB=+Z  RotationSequenceAxes=BaseAxes  RotationSequence=XYZ  RotationSequenceAngles=[0, 0, 0]  RotationSequenceAnglesUnits=rad  RotationMatrix=[1 0 0; 0 1 0; 0 0 1]
  ReferenceFrame : sm_lib/Frames and Transforms/Reference Frame
  Visual : sm_lib/Body Elements/File Solid  ExtGeomFileName=Brazo4_SLDASM/meshes/link_5.STL  UnitType=Custom  ExtGeomFileUnits=m  StepReaderType=HEX  ExportConvexHullGeometry=off  InertiaType=Custom  Mass=0  MassUnits=kg  CenterOfMass=[0, 0, 0]  CenterOfMassUnits=m  MomentsOfInertia=[0, 0, 0]  MomentsOfInertiaUnits=kg*m^2  ProductsOfInertia=[0, 0, 0]  ProductsOfInertiaUnits=kg*m^2  BasedOnType=DensityFromFile  Density=1000  DensityUnits=kg/m^3  DoExposeReferenceFrame=on  SerializedFrames=<Frames/>  GraphicType=FromGeometry  MarkerShape=Sphere  MarkerSize=10  GraphicVisPropType=SimpleVisualProperties  GraphicDiffuseColor=[0.77647, 0.75686, 0.73725]  GraphicSpecularColor=[0.5 0.5 0.5 1.0]  GraphicAmbientColor=[0.15 0.15 0.15 1.0]  GraphicEmissiveColor=[0.0 0.0 0.0 1.0]  GraphicShininess=75  GraphicOpacity=1
  VisualOriginTransform : sm_lib/Frames and Transforms/Rigid Transform  TranslationMethod=Cartesian  TranslationStandardOffset=0  TranslationLengthUnit=m  TranslationStandardAxis=+Z  TranslationCartesianOffset=[0, 0, 0]  TranslationROffset=0  TranslationROffsetUnits=m  TranslationZOffset=0  TranslationZOffsetUnits=m  TranslationThetaOffset=0  TranslationThetaOffsetUnits=deg  RotationMethod=RotationSequence  RotationAngleUnits=deg  RotationStandardAxis=+Z  RotationAngle=0.0  RotationArbitraryAxis=[0 0 1]  FollAlignAxisA=+X  BaseAlignAxisA=+Y  FollAlignAxisB=+Y  BaseAlignAxisB=+Z  RotationSequenceAxes=BaseAxes  RotationSequence=XYZ  RotationSequenceAngles=[0, 0, 0]  RotationSequenceAnglesUnits=rad  RotationMatrix=[1 0 0; 0 1 0; 0 0 1]
  end_effector_joint_OriginTransform : sm_lib/Frames and Transforms/Rigid Transform  TranslationMethod=Cartesian  TranslationStandardOffset=0  TranslationLengthUnit=m  TranslationStandardAxis=+Z  TranslationCartesianOffset=[0, 0, 0.1005]  TranslationROffset=0  TranslationROffsetUnits=m  TranslationZOffset=0  TranslationZOffsetUnits=m  TranslationThetaOffset=0  TranslationThetaOffsetUnits=deg  RotationMethod=RotationSequence  RotationAngleUnits=deg  RotationStandardAxis=+Z  RotationAngle=0.0  RotationArbitraryAxis=[0 0 1]  FollAlignAxisA=+X  BaseAlignAxisA=+Y  FollAlignAxisB=+Y  BaseAlignAxisB=+Z  RotationSequenceAxes=BaseAxes  RotationSequence=XYZ  RotationSequenceAngles=[0, 0, 0.045381]  RotationSequenceAnglesUnits=rad  RotationMatrix=[1 0 0; 0 1 0; 0 0 1]
  joint4_AxisInvTransform : sm_lib/Frames and Transforms/Rigid Transform  TranslationMethod=Cartesian  TranslationStandardOffset=0  TranslationLengthUnit=m  TranslationStandardAxis=+Z  TranslationCartesianOffset=[0, 0, 0]  TranslationROffset=0  TranslationROffsetUnits=m  TranslationZOffset=0  TranslationZOffsetUnits=m  TranslationThetaOffset=0  TranslationThetaOffsetUnits=deg  RotationMethod=ArbitraryAxis  RotationAngleUnits=rad  RotationStandardAxis=+Z  RotationAngle=0  RotationArbitraryAxis=[1, 0, 0]  FollAlignAxisA=+X  BaseAlignAxisA=+Y  FollAlignAxisB=+Y  BaseAlignAxisB=+Z  RotationSequenceAxes=FollowerAxes  RotationSequence=XYX  RotationSequenceAngles=[0 0 0]  RotationSequenceAnglesUnits=deg  RotationMatrix=[1 0 0; 0 1 0; 0 0 1]
  F : PMIOPort  Side=Left
  F1 : PMIOPort  Port=2  Side=Right
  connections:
  Inertia/RConn1 -- InertiaOriginTransform/RConn1
  ReferenceFrame/RConn1 -- InertiaOriginTransform/LConn1 -- VisualOriginTransform/LConn1 -- end_effector_joint_OriginTransform/LConn1 -- joint4_AxisInvTransform/LConn1
  Visual/RConn1 -- VisualOriginTransform/RConn1
  end_effector_joint_OriginTransform/RConn1 -- F1/RConn1
  joint4_AxisInvTransform/RConn1 -- F/RConn1

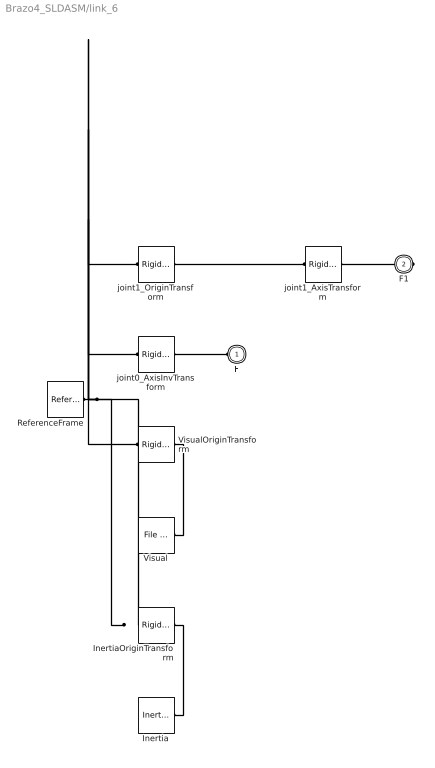
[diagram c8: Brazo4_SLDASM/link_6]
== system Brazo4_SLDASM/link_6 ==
  Inertia : sm_lib/Body Elements/Inertia  InertiaType=Custom  Mass=40.085  MassUnits=kg  CenterOfMass=[0, 0, 0]  CenterOfMassUnits=m  MomentsOfInertia=[0.14011, 0.15124, 0.16589]  MomentsOfInertiaUnits=kg*m^2  ProductsOfInertia=[-5.1752e-17, 1.3296e-17, 1.589e-18]  ProductsOfInertiaUnits=kg*m^2  GraphicType=None  MarkerShape=Inertia  MarkerSize=20  GraphicVisPropType=SimpleVisualProperties  GraphicDiffuseColor=[0.5 0.5 0.5]  GraphicSpecularColor=[0.5 0.5 0.5 1.0]  GraphicAmbientColor=[0.15 0.15 0.15 1.0]  GraphicEmissiveColor=[0.0 0.0 0.0 1.0]  GraphicShininess=75  GraphicOpacity=1.0
  InertiaOriginTransform : sm_lib/Frames and Transforms/Rigid Transform  TranslationMethod=Cartesian  TranslationStandardOffset=0  TranslationLengthUnit=m  TranslationStandardAxis=+Z  TranslationCartesianOffset=[2.7731e-17, 2.4685e-06, 0.28325]  TranslationROffset=0  TranslationROffsetUnits=m  TranslationZOffset=0  TranslationZOffsetUnits=m  TranslationThetaOffset=0  TranslationThetaOffsetUnits=deg  RotationMethod=RotationSequence  RotationAngleUnits=deg  RotationStandardAxis=+Z  RotationAngle=0.0  RotationArbitraryAxis=[0 0 1]  FollAlignAxisA=+X  BaseAlignAxisA=+Y  FollAlignAxisB=+Y  BaseAlignAxisB=+Z  RotationSequenceAxes=BaseAxes  RotationSequence=XYZ  RotationSequenceAngles=[0, 0, 0]  RotationSequenceAnglesUnits=rad  RotationMatrix=[1 0 0; 0 1 0; 0 0 1]
  ReferenceFrame : sm_lib/Frames and Transforms/Reference Frame
  Visual : sm_lib/Body Elements/File Solid  ExtGeomFileName=Brazo4_SLDASM/meshes/link_1.STL  UnitType=Custom  ExtGeomFileUnits=m  StepReaderType=HEX  ExportConvexHullGeometry=off  InertiaType=Custom  Mass=0  MassUnits=kg  CenterOfMass=[0, 0, 0]  CenterOfMassUnits=m  MomentsOfInertia=[0, 0, 0]  MomentsOfInertiaUnits=kg*m^2  ProductsOfInertia=[0, 0, 0]  ProductsOfInertiaUnits=kg*m^2  BasedOnType=DensityFromFile  Density=1000  DensityUnits=kg/m^3  DoExposeReferenceFrame=on  SerializedFrames=<Frames/>  GraphicType=FromGeometry  MarkerShape=Sphere  MarkerSize=10  GraphicVisPropType=SimpleVisualProperties  GraphicDiffuseColor=[0.77647, 0.75686, 0.73725]  GraphicSpecularColor=[0.5 0.5 0.5 1.0]  GraphicAmbientColor=[0.15 0.15 0.15 1.0]  GraphicEmissiveColor=[0.0 0.0 0.0 1.0]  GraphicShininess=75  GraphicOpacity=1
  VisualOriginTransform : sm_lib/Frames and Transforms/Rigid Transform  TranslationMethod=Cartesian  TranslationStandardOffset=0  TranslationLengthUnit=m  TranslationStandardAxis=+Z  TranslationCartesianOffset=[0, 0, 0]  TranslationROffset=0  TranslationROffsetUnits=m  TranslationZOffset=0  TranslationZOffsetUnits=m  TranslationThetaOffset=0  TranslationThetaOffsetUnits=deg  RotationMethod=RotationSequence  RotationAngleUnits=deg  RotationStandardAxis=+Z  RotationAngle=0.0  RotationArbitraryAxis=[0 0 1]  FollAlignAxisA=+X  BaseAlignAxisA=+Y  FollAlignAxisB=+Y  BaseAlignAxisB=+Z  RotationSequenceAxes=BaseAxes  RotationSequence=XYZ  RotationSequenceAngles=[0, 0, 0]  RotationSequenceAnglesUnits=rad  RotationMatrix=[1 0 0; 0 1 0; 0 0 1]
  joint0_AxisInvTransform : sm_lib/Frames and Transforms/Rigid Transform  TranslationMethod=Cartesian  TranslationStandardOffset=0  TranslationLengthUnit=m  TranslationStandardAxis=+Z  TranslationCartesianOffset=[0, 0, 0]  TranslationROffset=0  TranslationROffsetUnits=m  TranslationZOffset=0  TranslationZOffsetUnits=m  TranslationThetaOffset=0  TranslationThetaOffsetUnits=deg  RotationMethod=ArbitraryAxis  RotationAngleUnits=rad  RotationStandardAxis=+Z  RotationAngle=0  RotationArbitraryAxis=[1, 0, 0]  FollAlignAxisA=+X  BaseAlignAxisA=+Y  FollAlignAxisB=+Y  BaseAlignAxisB=+Z  RotationSequenceAxes=FollowerAxes  RotationSequence=XYX  RotationSequenceAngles=[0 0 0]  RotationSequenceAnglesUnits=deg  RotationMatrix=[1 0 0; 0 1 0; 0 0 1]
  joint1_AxisTransform : sm_lib/Frames and Transforms/Rigid Transform  TranslationMethod=Cartesian  TranslationStandardOffset=0  TranslationLengthUnit=m  TranslationStandardAxis=+Z  TranslationCartesianOffset=[0, 0, 0]  TranslationROffset=0  TranslationROffsetUnits=m  TranslationZOffset=0  TranslationZOffsetUnits=m  TranslationThetaOffset=0  TranslationThetaOffsetUnits=deg  RotationMethod=ArbitraryAxis  RotationAngleUnits=rad  RotationStandardAxis=+Z  RotationAngle=0  RotationArbitraryAxis=[1, 0, 0]  FollAlignAxisA=+X  BaseAlignAxisA=+Y  FollAlignAxisB=+Y  BaseAlignAxisB=+Z  RotationSequenceAxes=FollowerAxes  RotationSequence=XYX  RotationSequenceAngles=[0 0 0]  RotationSequenceAnglesUnits=deg  RotationMatrix=[1 0 0; 0 1 0; 0 0 1]
  joint1_OriginTransform : sm_lib/Frames and Transforms/Rigid Transform  TranslationMethod=Cartesian  TranslationStandardOffset=0  TranslationLengthUnit=m  TranslationStandardAxis=+Z  TranslationCartesianOffset=[0, 0, 0.35051]  TranslationROffset=0  TranslationROffsetUnits=m  TranslationZOffset=0  TranslationZOffsetUnits=m  TranslationThetaOffset=0  TranslationThetaOffsetUnits=deg  RotationMethod=RotationSequence  RotationAngleUnits=deg  RotationStandardAxis=+Z  RotationAngle=0.0  RotationArbitraryAxis=[0 0 1]  FollAlignAxisA=+X  BaseAlignAxisA=+Y  FollAlignAxisB=+Y  BaseAlignAxisB=+Z  RotationSequenceAxes=BaseAxes  RotationSequence=XYZ  RotationSequenceAngles=[1.5708, 0, 1.5708]  RotationSequenceAnglesUnits=rad  RotationMatrix=[1 0 0; 0 1 0; 0 0 1]
  F : PMIOPort  Side=Left
  F1 : PMIOPort  Port=2  Side=Right
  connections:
  Inertia/RConn1 -- InertiaOriginTransform/RConn1
  ReferenceFrame/RConn1 -- InertiaOriginTransform/LConn1 -- VisualOriginTransform/LConn1 -- joint0_AxisInvTransform/LConn1 -- joint1_OriginTransform/LConn1
  Visual/RConn1 -- VisualOriginTransform/RConn1
  joint0_AxisInvTransform/RConn1 -- F/RConn1
  joint1_AxisTransform/RConn1 -- F1/RConn1
  joint1_AxisTransform/LConn1 -- joint1_OriginTransform/RConn1
